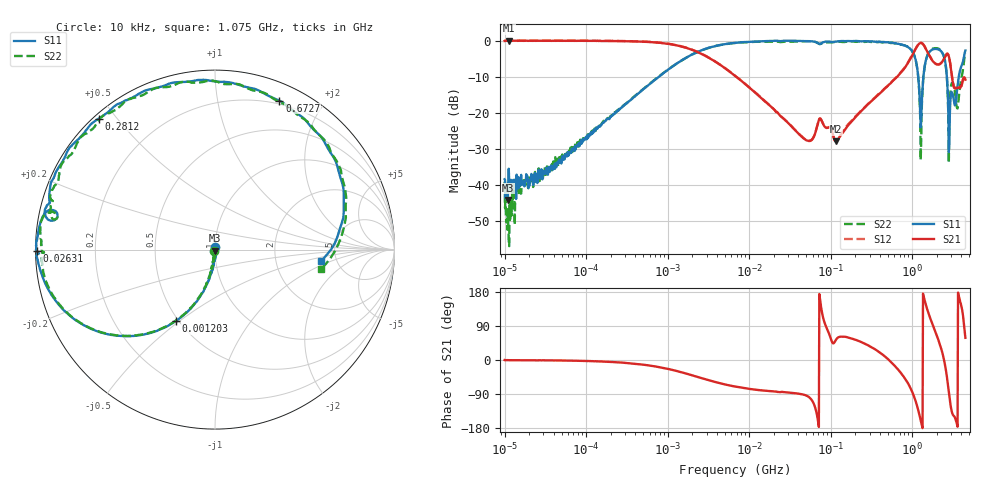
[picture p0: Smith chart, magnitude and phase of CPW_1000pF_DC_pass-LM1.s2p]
!Siglent Technologies,SNA5004A,SNA5XCED5R0097,V1.0.0.2.10.R9
!Date: 2024-10-29 17:23:34
!Data & Calibration Information:
!Freq	S11:F2(ON)	S21:F2(ON)	S12:F2(ON)	S22:F2(ON)
# Hz S DB R 50
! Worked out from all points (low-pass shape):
!   1001 points, 10 kHz to 4.5 GHz, reference 50 ohm
!   highest |S21| = -0.01 dB at 11.39 kHz (marker M1); lowest = -28.0 dB at 116.1 MHz (marker M2)
!   |S21| within 3 dB of the highest: start of sweep to 2.244 MHz; 1.061 GHz to 1.529 GHz (468 MHz wide, 36.1 % of centre)
!   lowest |S11| = -44.2 dB at 10.95 kHz (marker M3), VSWR 1.01, Z = 50 - j0.614 ohm
!   |S11| at or under -10 dB: start of sweep to 783.2 kHz; 1.186 GHz to 1.374 GHz (187.9 MHz wide, 14.7 % of centre); 2.666 GHz to 3.731 GHz (1.065 GHz wide, 33.3 % of centre)
!   |S22| runs from -57.1 to -0.1 dB; largest |S21 - S12| = 0.017
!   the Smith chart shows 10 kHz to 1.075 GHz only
!   S11 on the Smith chart (normalised r, x): 10 kHz: 1.00, +0.02; 1.203 MHz: 0.48, -0.48; 26.31 MHz: 0.00, -0.00; 281.2 MHz: 0.01, +0.45; 672.7 MHz: 0.16, +1.51; 1.075 GHz: 3.80, -0.75
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10000  -38.49 100.2  -0.09 -0.1  -0.01 -0.1  -39.19 -124.4
10953.99  -44.24 -89.3  -0.03 -0.4  0.01 -0.4  -46.79 -77.1
11390.22  -39.12 -80.0  -0.01 -0.5  0.02 -0.5  -57.08 -55.0
14397.59  -39.59 -95.7  -0.07 -0.6  -0.01 -0.7  -40.35 -124.3
87919.76  -28.63 -90.9  -0.06 -2.2  -0.01 -2.3  -27.95 -95.8
772988.4  -10.07 -110.0  -0.59 -18.5  -0.54 -18.6  -10.03 -110.4
1203323  -6.86 -118.8  -1.18 -27.3  -1.14 -27.4  -6.84 -119.1
6708204  -0.61 -162.1  -9.77 -70.0  -9.72 -70.1  -0.66 -162.0
2.631441e7  -0.05 -179.4  -21.60 -84.6  -21.57 -84.9  -0.33 -179.3
5.897837e7  -0.19 169.3  -27.54 -106.5  -27.44 -106.7  -0.20 169.7
1.160539e8  -0.26 162.2  -28.01 53.1  -27.82 53.1  -0.30 162.1
2.812408e8  -0.21 131.6  -17.85 40.1  -17.77 40.0  -0.24 131.0
5.185364e8  -0.52 91.7  -12.22 0.1  -12.16 0.3  -0.51 90.9
6.727342e8  -0.87 66.7  -9.77 -25.2  -9.67 -24.8  -0.95 65.8
1.074878e9  -4.49 -6.1  -2.75 -101.1  -2.71 -100.8  -4.43 -10.5
1.273066e9  -24.12 3.7  -0.65 -158.9  -0.60 -158.5  -33.19 -52.2
1.588384e9  -3.54 29.5  -3.76 123.1  -3.69 123.6  -3.45 32.8
1.881253e9  -2.34 -12.3  -6.23 80.2  -6.16 80.7  -2.11 -11.0
2.257315e9  -2.89 -62.2  -6.28 32.4  -6.22 33.1  -2.85 -61.8
2.779993e9  -20.42 177.1  -3.99 -75.1  -3.91 -74.4  -21.40 -179.4
3.701812e9  -10.47 49.4  -13.11 172.0  -13.08 173.2  -16.62 87.3
4.5e9  -2.75 -31.1  -10.85 58.5  -10.93 56.3  -3.37 -17.7
